TYPE LstBIASUnit :
STRUCT
	BIAS_UnitName: STRING;
	BIAS_RFPower: INT;
	BIAS_TuneCapPreset: INT;
	BIAS_LoadCapPreset: INT;
	BIAS_AutoTuneCapPreset: INT;
	BIAS_AutoLoadCapPreset: INT;
	BIAS_MaxReflectedPower: INT;
	BIAS_GeneratorMode: STRING;
	BIAS_PulseRateFreq: INT;
	BIAS_PulseDutyCycle: INT;
	BIAS_EnableRamp: BOOL;
	BIAS_TargetMode: STRING;
	BIAS_TargetBiasRFPower: INT;
END_STRUCT
END_TYPE
